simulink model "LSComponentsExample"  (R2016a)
settings: Solver=VariableStepAuto  StartTime=0.0  StopTime=Tf  RelTol=1e-7  AbsTol=1e-6
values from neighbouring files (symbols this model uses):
  Gden = [1 0]    [Section6p3_TradeoffsExample.m]    (also in Section6p5_LSComponentsExample.m = [1 2])
  Gnum = 1    [Section6p3_TradeoffsExample.m]    (also in Section6p5_LSComponentsExample.m = 5)
  Kden = [1 wbar]    [Section6p5_LSComponentsExample.m]
  Knum = wbar    (= 10)    [Section6p5_LSComponentsExample.m]

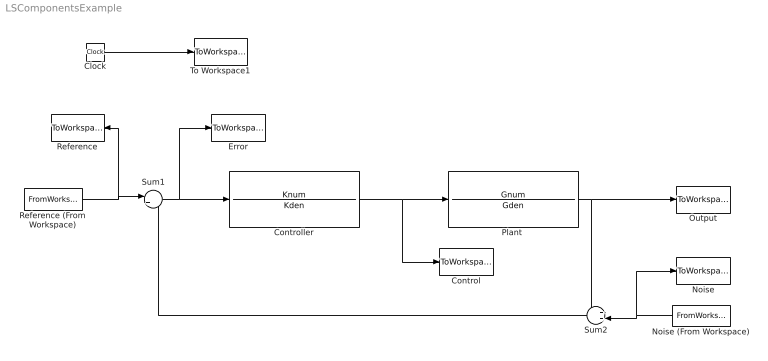
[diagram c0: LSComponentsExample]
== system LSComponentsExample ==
  Clock : Clock
  Control : ToWorkspace  VariableName=u  SampleTime=-1
  Controller : TransferFcn  Numerator=Knum  Denominator=Kden
  Error : ToWorkspace  VariableName=e  SampleTime=-1
  Noise : ToWorkspace  VariableName=n  SampleTime=-1
  Noise (From Workspace) : FromWorkspace  VariableName=nData  SampleTime=0
  Output : ToWorkspace  VariableName=y  SampleTime=-1
  "Plant " : TransferFcn  Numerator=Gnum  Denominator=Gden
  Reference : ToWorkspace  VariableName=r  SampleTime=-1
  Reference (From Workspace) : FromWorkspace  VariableName=rData  SampleTime=0
  Sum1 : Sum  Inputs=|+-
  Sum2 : Sum  Inputs=++|
  To Workspace1 : ToWorkspace  VariableName=t  SampleTime=-1
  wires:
  Clock/1 -> To Workspace1/1
  Controller/1 -> "Plant "/1, Control/1
  "Plant "/1 -> Sum2/1, Output/1
  Sum1/1 -> Controller/1, Error/1
  Sum2/1 -> Sum1/2
  Reference (From Workspace)/1 -> Reference/1, Sum1/1
  Noise (From Workspace)/1 -> Noise/1, Sum2/2
